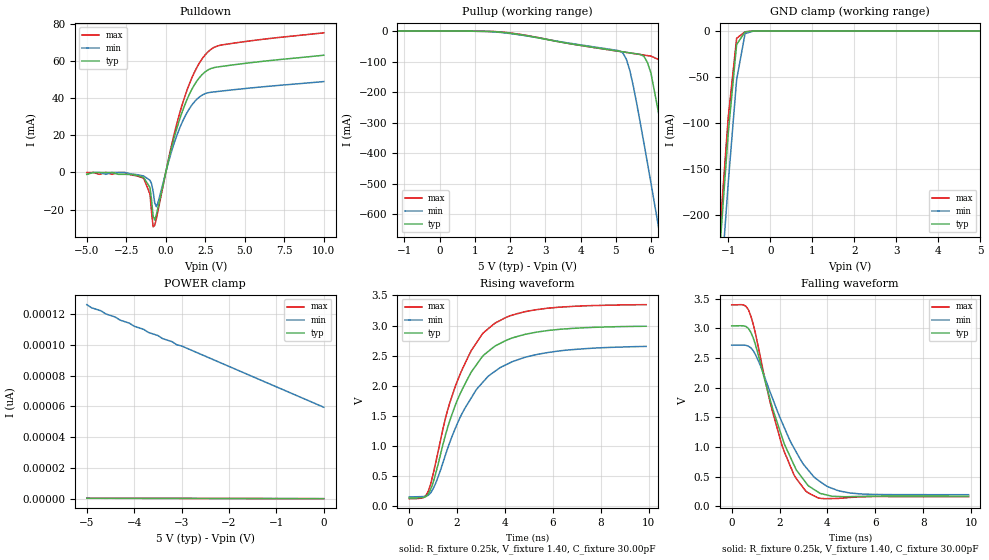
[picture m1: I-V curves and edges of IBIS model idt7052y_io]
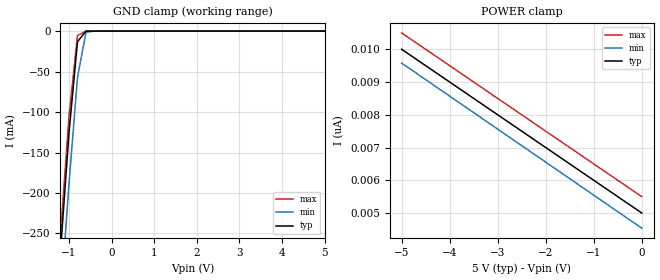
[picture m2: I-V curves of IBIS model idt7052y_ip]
| IBIS file 7052y.ibs created by s2ibis2 version 1.1
| North Carolina State University Electronics Research Laboratory  1995
[IBIS ver]   2.1
[File name]   7052pq.ibs
[File Rev]   1.0
[Date]   03/24/98
[Source]   Integrated Device Technology, Inc.
[Notes]   1.Temperatures: typ=25C, min=100C, max=0C 2.Cemos8 5vv
   process. 3.RRmp rates based on 50 ohm load.
[Disclaimer] Integrated Device Technology, Inc. ("IDT") hereby grants the
   user of this IBIS model a non-exclusive, nontransferable
   license to use this IBIS model under the following terms. The
   user is granted this license only to use the IBIS model and is
   not granted rights to sell, copy (except as needed to run the
   IBIS model), rent, lease or sub-license the IBIS model in
   whole or in part, or in modified form to anyone. The User may
   modify the IBIS model to suit its specific applications, but
   rights to derivative works and such modifications shall belong
   to IDT. This IBIS model is provided on an AS IS" basis and IDT
   makes absolutely no warranty with respect to the information
   contained herein. IDT DISCLAIMS AND CUSTOMER WAIVES ALL
   WARRANTIES, EXPRESS AND IMPLIED, INCLUDING WARRANTIES OF
   MERCHANTABILITY AND FITNESS FOR A PARTICULAR PURPOSE. THE
   ENTIRE RISK AS TO QUALITY AND PERFORMANCE IS WITH THE USER
   ACCORDINGLY, IN NO EVENT SHALL IDT BE LIABLE FOR ANY DIRECT OR
   INDIRECT DAMAGES, WHETHER IN CONTRACT OR TORT, INCLUDING ANY
   LOST PROFITS OR OTHER INCIDENTAL, CONSEQUENTIAL, EXEMPLARY, OR
   PUNITIVE DAMAGES ARISING OUT OF THE USE OR APPLICATION OF THE
   IBIS model. Further, IDT reserves the right to make changes
   without notice to any product herein to improve reliability,
   function, or design. IDT does not convey any license under
   patent rights or any other intellectual property rights,
   including those of third parties. IDT is not obligated to
   provide maintenance or support for the licensed IBIS model.
[Copyright]   Copyright 1997, Integrated Device Technology, Inc. all rights
   reserved
|   Component 7052y
[Component]   7052y
[Manufacturer]   Integrated Device Technology
[Package]
| variable   typ   min   max
R_pkg   200.00m   100.00m   300.00m
L_pkg   10.00nH   9.00nH   12.00nH
C_pkg   0.20pF   0.10pF   0.30pF
[Pin]  signal_name   model_name   R_pin L_pin C_pin
1   nc   nc
2   a0p2   idt7052y_ip
3   a1p2   idt7052y_ip
4   a2p2   idt7052y_ip
5   a3p2   idt7052y_ip
6   a4p2   idt7052y_ip
7   a5p2   idt7052y_ip
8   a6p2   idt7052y_ip
9   nc   nc
10   a10p2   idt7052y_ip
11   a7p2   idt7052y_ip
12   a8p2   idt7052y_ip
13   a9p2   idt7052y_ip
14   nc   nc
15   rwlp2   idt7052y_ip
16   celp2   idt7052y_ip
17   nc   nc
18   nc   nc
19   oelp2   idt7052y_ip
20   busylp2   idt7052y_ip
21   nc   nc
22   a0p1   idt7052y_ip
23   a1p1   idt7052y_ip
24   a2p1   idt7052y_ip
25   a3p1   idt7052y_ip
26   a4p1   idt7052y_ip
27   a5p1   idt7052y_ip
28   a6p1   idt7052y_ip
29   nc   nc
30   a10p1   idt7052y_ip
31   vcc   POWER
32   a7p1   idt7052y_ip
33   a8p1   idt7052y_ip
34   a9p1   idt7052y_ip
35   nc   nc
36   celp1   idt7052y_ip
37   rwlp1   idt7052y_ip
38   oelp1   idt7052y_ip
39   busylp1   idt7052y_ip
40   nc   nc
41   io0p1   idt7052y_io
42   io1p1   idt7052y_io
43   io2p1   idt7052y_io
44   io3p1   idt7052y_io
45   gnd   GND
46   nc   nc
47   io4p1   idt7052y_io
48   io5p1   idt7052y_io
49   nc   nc
50   nc   nc
51   nc   nc
52   io6p1   idt7052y_io
53   io7p1   idt7052y_io
54   nc   nc
55   vcc   POWER
56   nc   nc
57   io0p2   idt7052y_io
58   io1p2   idt7052y_io
59   io2p2   idt7052y_io
60   gnd   GND
61   io3p2   idt7052y_io
62   io4p2   idt7052y_io
63   io5p2   idt7052y_io
64   vcc   POWER
65   io6p2   idt7052y_io
66   io7p2   idt7052y_io
67   nc   nc
68   io0p3   idt7052y_io
69   io1p3   idt7052y_io
70   vcc   POWER
71   io2p3   idt7052y_io
72   io3p3   idt7052y_io
73   io4p3   idt7052y_io
74   gnd   GND
75   nc   nc
76   io5p3   idt7052y_io
77   io6p3   idt7052y_io
78   io7p3   idt7052y_io
79   nc   nc
80   vcc   POWER
81   io0p4   idt7052y_io
82   io1p4   idt7052y_io
83   nc   nc
84   nc   nc
85   nc   nc
86   io2p4   idt7052y_io
87   io3p4   idt7052y_io
88   io4p4   idt7052y_io
89   gnd   GND
90   io5p4   idt7052y_io
91   io6p4   idt7052y_io
92   io7p4   idt7052y_io
93   nc   nc
94   gnd   GND
95   nc   nc
96   busylp4   idt7052y_ip
97   oelp4   idt7052y_ip
98   rwlp4   idt7052y_ip
99   celp4   idt7052y_ip
100   nc   nc
101   a9p4   idt7052y_ip
102   a8p4   idt7052y_ip
103   a7p4   idt7052y_ip
104   gnd   GND
105   a10p4   idt7052y_ip
106   nc   nc
107   a6p4   idt7052y_ip
108   a5p4   idt7052y_ip
109   a4p4   idt7052y_ip
110   a3p4   idt7052y_ip
111   a2p4   idt7052y_ip
112   a1p4   idt7052y_ip
113   a0p4   idt7052y_ip
114   nc   nc
115   busylp3   idt7052y_ip
116   nc   nc
117   nc   nc
118   rwlp3   idt7052y_ip
119   celp3   idt7052y_ip
120   oelp3   idt7052y_ip
121   nc   nc
122   a9p3   idt7052y_ip
123   a8p3   idt7052y_ip
124   a7p3   idt7052y_ip
125   a10p3   idt7052y_ip
126   a6p3   idt7052y_ip
127   a5p3   idt7052y_ip
128   a4p3   idt7052y_ip
129   a3p3   idt7052y_ip
130   a2p3   idt7052y_ip
131   a1p3   idt7052y_ip
132   a0p3   idt7052y_ip
| Models and submodels in the file (2): idt7052y_io (I/O), idt7052y_ip (Input)
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|   Model idt7052y_io
[Model]   idt7052y_io
Model_type   I/O
Polarity   Inverting
Enable   Active-High
Vinl =  0.000V
Vinh =  5.000V
Vmeas =  1.500V
C_comp   3.00pF   NA   NA
[Temperature Range]   25.00   100.00   0.000
[Voltage Range]   5.00V   4.50V   5.50V
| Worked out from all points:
|   slope of the pulldown table from 0 to 0.75 V, typ, clamps not added: 29.8 ohm
|   slope of the pullup table from 0 to 0.75 V, typ, clamps not added: 5.4 kohm
|   GND clamp passes 1 mA (typ) near -0.60 V on its own axis
|   rising waveform, R_fixture 0.25k, V_fixture 1.40, C_fixture 30.00pF: 20-80 % time 1.72ns typ, 1.94ns min, 1.66ns max; typ from 0.133 V to 2.99 V
|   falling waveform, R_fixture 0.25k, V_fixture 1.40, C_fixture 30.00pF: 20-80 % time 1.38ns typ, 1.67ns min, 1.24ns max; typ from 3.04 V to 0.173 V
[Pulldown]
| voltage   I(typ)   I(min)   I(max)
-5V       -1mA       -1mA       0A
-1.4V     -2.7mA     -1.9mA     -3.1mA
-1V       -8.1mA     -4.2mA     -11.71mA
-800mV    -23.62mA   -10.2mA    -29.36mA
-600mV    -22.92mA   -18.47mA   -25.06mA
-500mV    -19.25mA   -16.48mA   -20.98mA
300mV     11.1mA     9.447mA    12.19mA
1V        31.75mA    26.37mA    35.49mA
1.7V      45.65mA    36.94mA    52.02mA
2.5V      54.37mA    42.57mA    63.55mA
3.5V      57.22mA    43.93mA    68.79mA
10V       63.3mA     49.09mA    75.4mA
[Pullup]
| voltage   I(typ)   I(min)   I(max)
-5V       0A         1.1pA      -14.2fA
1.6V      -2.448mA   -3.262mA   -2.012mA
5.1V      -66.29mA   -64.85mA   -66.71mA
5.3V      -69.72mA   -91.99mA   -70.16mA
5.4V      -71.44mA   -129mA     -71.87mA
5.8V      -82.54mA   -367mA     -78.71mA
6V        -138mA     -498mA     -82.12mA
6.4V      -379mA     -767mA     -103mA
6.8V      -647mA     -1.039A    -297mA
7.2V      -919mA     -1.313A    -563mA
7.6V      -1.193A    -1.588A    -835mA
10V       -2.855A    -3.249A    -2.493A
[GND_clamp]
| voltage   I(typ)   I(min)   I(max)
-5V       -2.848A    -2.896A    -2.833A
-1.2V     -237mA     -292mA     -219mA
-1V       -111mA     -165mA     -93.89mA
-800mV    -14.56mA   -52.79mA   -7.9mA
-600mV    -913uA     -2.906mA   -830uA
-400mV    -6.881nA   -19.42uA   -410pA
5V        249fA      66.14pA    242fA
[POWER_clamp]
| voltage   I(typ)   I(min)   I(max)
-5V       554fA      126pA      554fA
-4.9V     526fA      124pA      540fA
-4.4V     512fA      118pA      512fA
-4.3V     512fA      116pA      512fA
-4.1V     497fA      114pA      497fA
-4V       483fA      112pA      497fA
-3.8V     469fA      110pA      483fA
-3.7V     469fA      108pA      483fA
-3.5V     455fA      106pA      455fA
-3.1V     426fA      100pA      455fA
-3V       426fA      99.23pA    441fA
0V        249fA      59.53pA    270fA
[Ramp]
| variable   typ   min   max
dV/dt_r   0.99/0.35n   0.83/0.46n   1.14/0.32n
dV/dt_f   1.60/0.62n   1.27/0.78n   1.87/0.54n
R_load = 50.00
[Rising Waveform]
R_fixture = 0.25k
V_fixture = 1.40
C_fixture = 30.00pF
R_dut = 30.00m
L_dut = 9.00nH
C_dut = 0.35pF
| time   V(typ)   V(min)   V(max)
0s        133mV      153mV      122mV
600ps     142mV      158mV      141mV
800ps     204mV      180mV      250mV
1ns       391mV      289mV      533mV
1.5ns     1.161V     832mV      1.438V
2ns       1.751V     1.361V     2.068V
2.6ns     2.232V     1.802V     2.59V
3.5ns     2.634V     2.216V     3.014V
5.8ns     2.918V     2.552V     3.289V
9.9ns     2.988V     2.653V     3.347V
[Falling Waveform]
R_fixture = 0.25k
V_fixture = 1.40
C_fixture = 30.00pF
R_dut = 30.00m
L_dut = 9.00nH
C_dut = 0.35pF
| time   V(typ)   V(min)   V(max)
0s        3.04V      2.715V     3.394V
700ps     2.995V     2.697V     3.311V
1.2ns     2.416V     2.374V     2.515V
1.6ns     1.807V     1.933V     1.764V
2.1ns     1.172V     1.42V      1.03V
2.6ns     701mV      986mV      535mV
3.1ns     401mV      660mV      258mV
4ns       190mV      335mV      131mV
4.9ns     164mV      229mV      150mV
9.9ns     173mV      197mV      163mV
|   Model idt7052y_ip
[Model]   idt7052y_ip
Model_type   Input
Vinl =  0.800V
Vinh =  2.200V
Vmeas =  1.500V
C_comp   3.00pF   NA   NA
[Temperature Range]   25.00   100.00   0.000
[Voltage Range]   5.00V   4.50V   5.50V
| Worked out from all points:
|   GND clamp passes 1 mA (typ) near -0.61 V on its own axis
[GND_clamp]
| voltage   I(typ)   I(min)   I(max)
-5V       -3.321A    -3.376A    -3.303A
-1.2V     -273mA     -336mA     -252mA
-1V       -126mA     -189mA     -106mA
-800mV    -13.06mA   -57.24mA   -5.45mA
-600mV    -97.49uA   -1.45mA    -20.3uA
-400mV    -4.308nA   -2.066uA   -632pA
5V        5nA        5.041nA    5nA
[POWER_clamp]
| voltage   I(typ)   I(min)   I(max)
-5V       10nA       9.578nA    10.5nA
-4.8V     9.801nA    9.377nA    10.3nA
-4.4V     9.401nA    8.973nA    9.901nA
0V        5nA        4.537nA    5.5nA
